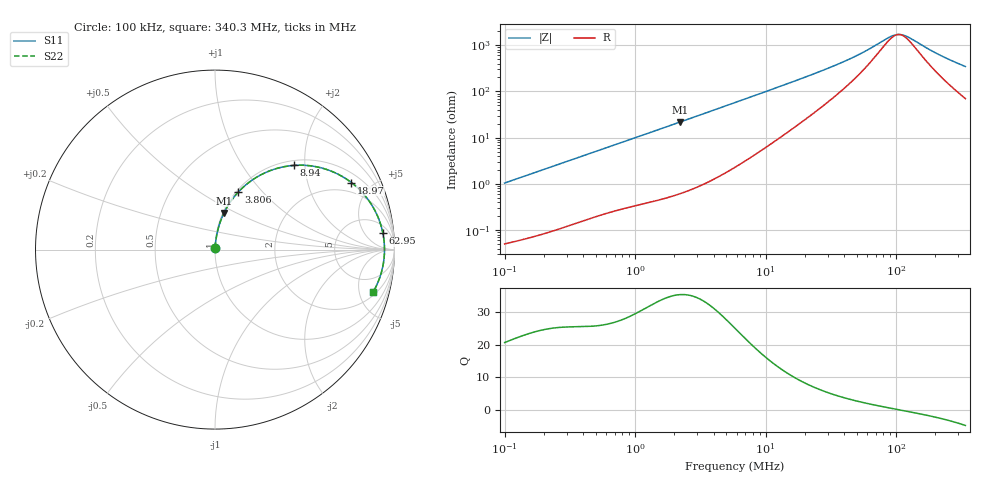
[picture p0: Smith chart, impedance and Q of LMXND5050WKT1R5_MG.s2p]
! LMXND5050WKT1R5_MG  S-PARAMETER MODEL  ( General Type )
! Model Generated by TAIYO YUDEN Corporation (https://www.yuden.co.jp/en/)
! Version 1.0
! TAIYO YUDEN Control No. 191023NI43SB-FBB
! Copyright(c) 2019 TAIYO YUDEN CO.,LTD. All Rights Reserved.
! Product Description (link to TY-COMPAS)
! https://ds.yuden.co.jp/TYCOMPAS/or/detail?pn=LMXND5050WKT1R5NMG&u=M
! Products Name : Inductors
! Characteristics :
!  Inductance : 1.5 uH , SRF(min) : 68 MHz , DC Resistance(max) : 0.0312 Ohm
!  Rated Current : Saturation :3350 mA , Temp Rise : 3200 mA (40 degC)
!  Case Size : 4.9 x 4.9 / 0.193 x 0.193 [mm/inch] , Thickness : 2 / 0.079 [mm/inch]
!  (Conditions: Temperature = 25 degC , DC Bias Current/Voltage = 0A / 0V)
! External Node Assignments :
!  1  o---GGG---o  2
! GND o---------o GND
! Frequency Range : 0.1MHz  -  340.31115MHz  [ 402 STEP ]
# MHz S RI R 50
! Freq[MHz].  S11 Real  S11 Imag  S21 Real  S21 Imag  S12 Real  S12 Imag  S22 Real  S22 Imag
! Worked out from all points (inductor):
!   401 points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, 100 kHz to 340.3 MHz, reference 50 ohm
!   read as one part in series: L = 1.65 uH near 104.2 kHz
!   highest Q = 35.4 at 2.198 MHz (marker M1), where L = 1.56 uH
!   self-resonance near 105.1 MHz
!   S11 on the Smith chart (normalised r, x): 100 kHz: 1.00, +0.02; 3.806 MHz: 1.02, +0.75; 8.94 MHz: 1.10, +1.76; 18.97 MHz: 1.44, +3.79; 62.95 MHz: 9, +15; 340.3 MHz: 2.40, -6.75
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0.1  0.000614 0.0104  0.9994 -0.0104  0.9994 -0.0104  0.000614 0.0104
0.390471  0.00312 0.0395  0.9969 -0.0395  0.9969 -0.0395  0.00312 0.0395
0.828491  0.00966 0.0816  0.9903 -0.0816  0.9903 -0.0816  0.00966 0.0816
1.524679  0.0263 0.1458  0.9737 -0.1458  0.9737 -0.1458  0.0263 0.1458
2.198432  0.0499 0.2041  0.9501 -0.2041  0.9501 -0.2041  0.0499 0.2041
3.806401  0.1302 0.3212  0.8698 -0.3212  0.8698 -0.3212  0.1302 0.3212
5.953437  0.2633 0.4207  0.7367 -0.4207  0.7367 -0.4207  0.2633 0.4207
8.940495  0.4404 0.4692  0.5596 -0.4692  0.5596 -0.4692  0.4404 0.4692
12.63183  0.6029 0.4524  0.3971 -0.4524  0.3971 -0.4524  0.6029 0.4524
18.96969  0.7602 0.3733  0.2398 -0.3733  0.2398 -0.3733  0.7602 0.3733
22.77862  0.8119 0.3272  0.1881 -0.3272  0.1881 -0.3272  0.8119 0.3272
29.66971  0.8667 0.259  0.1333 -0.259  0.1333 -0.259  0.8667 0.259
40.24933  0.9064 0.1852  0.0936 -0.1852  0.0936 -0.1852  0.9064 0.1852
51.37064  0.9255 0.1322  0.0745 -0.1322  0.0745 -0.1322  0.9255 0.1322
62.95234  0.9353 0.0918  0.0647 -0.0918  0.0647 -0.0918  0.9353 0.0918
88.94399  0.9435 0.029  0.0565 -0.029  0.0565 -0.029  0.9435 0.029
102.5473  0.9444 0.00429  0.0556 -0.00429  0.0556 -0.00429  0.9444 0.00429
108.9967  0.9444 -0.00627  0.0556 0.00627  0.0556 0.00627  0.9444 -0.00627
118.2312  0.944 -0.0204  0.056 0.0204  0.056 0.0204  0.944 -0.0204
213.203  0.9261 -0.1304  0.0739 0.1304  0.0739 0.1304  0.9261 -0.1304
277.7022  0.9054 -0.1879  0.0946 0.1879  0.0946 0.1879  0.9054 -0.1879
340.3111  0.8809 -0.2365  0.1191 0.2365  0.1191 0.2365  0.8809 -0.2365
